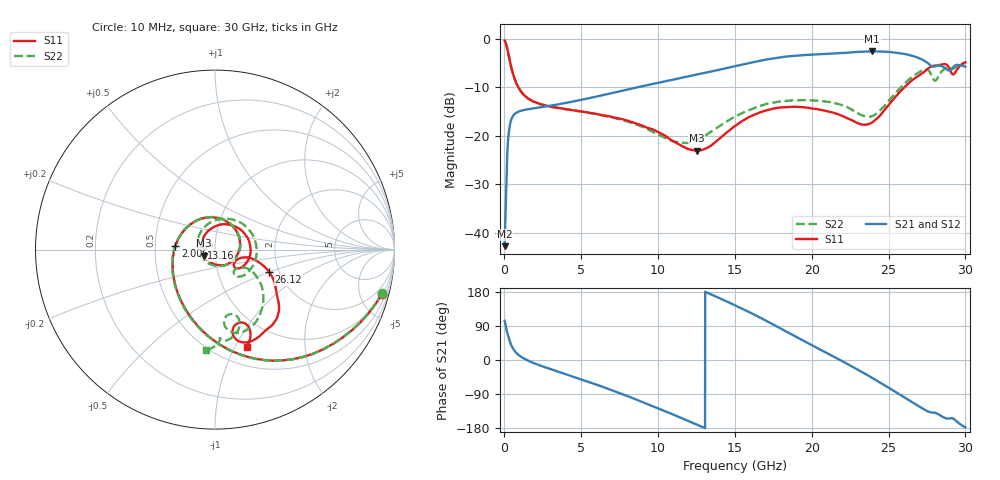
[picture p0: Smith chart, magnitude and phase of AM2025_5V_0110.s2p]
!Keysight Technologies,N5245B,MY58422270,A.16.20.02
!Date: Tuesday, July 14, 2026 01:05:04
!Correction: S11(C  2-Port  )
!S21(C  2-Port  )
!S12(C  2-Port  )
!S22(C  2-Port  )
!S2P File: Measurements: S11, S21, S12, S22:
# Hz S  dB  R 50
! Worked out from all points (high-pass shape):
!   3201 points, 10 MHz to 30 GHz, reference 50 ohm
!   highest |S21| = -2.59 dB at 23.94 GHz (marker M1); lowest = -42.8 dB at 10 MHz (marker M2)
!   |S21| within 3 dB of the highest: 15.09 GHz to 27.78 GHz (12.69 GHz wide, 59.2 % of centre); 29.28 GHz to 29.83 GHz (548.6 MHz wide, 1.86 % of centre)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
!   lowest |S11| = -23.1 dB at 12.5 GHz (marker M3), VSWR 1.15, Z = 44.1 - j3.06 ohm
!   |S11| at or under -10 dB: 904.8 MHz to 26.03 GHz (25.13 GHz wide, 187 % of centre)
!   |S22| runs from -21.5 to -0.3 dB; largest |S21 - S12| = 0.017
!   S11 on the Smith chart (normalised r, x): 10 MHz: 1.16, -7.56; 2.006 GHz: 0.64, +0.03; 13.16 GHz: 0.86, +0.02; 26.12 GHz: 1.77, -0.49; 30 GHz: 0.69, -1.12
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1e7  -0.34 -14.7  -42.79 103.5  -32.97 80.0  -0.34 -14.5
2.536688e8  -3.11 -62.2  -20.24 62.0  -20.22 62.0  -3.13 -62.6
4.317344e8  -5.75 -89.2  -16.79 40.3  -16.79 40.3  -5.77 -89.8
9.003281e8  -9.97 -131.1  -15.04 14.0  -15.04 14.0  -10.01 -132.3
2.006209e9  -13.09 174.5  -14.29 -9.7  -14.29 -9.7  -13.15 172.1
5.014581e9  -15.00 87.6  -12.58 -51.3  -12.57 -51.4  -15.01 82.2
7.535616e9  -16.48 24.5  -10.81 -88.0  -10.81 -88.0  -16.64 16.5
1.000979e10  -19.25 -44.6  -9.07 -127.4  -9.08 -127.5  -19.75 -59.0
1.250271e10  -23.08 -150.6  -7.38 -170.0  -7.37 -170.1  -20.92 -167.2
1.315874e10  -22.54 172.9  -6.94 178.3  -6.93 178.2  -19.78 163.2
1.5005e10  -17.99 93.4  -5.65 144.3  -5.65 144.3  -16.04 95.3
1.776033e10  -14.26 18.3  -3.90 87.8  -3.90 87.8  -13.01 23.9
2.000958e10  -14.37 -20.8  -3.26 39.1  -3.26 39.0  -12.71 -17.8
2.209014e10  -16.07 -41.7  -2.91 -5.3  -2.91 -5.3  -13.82 -47.5
2.39364e10  -17.23 -22.9  -2.59 -47.2  -2.60 -47.2  -15.94 -39.9
2.500479e10  -13.66 -13.4  -2.70 -73.1  -2.70 -73.2  -12.82 -30.1
2.612004e10  -9.74 -22.4  -3.16 -100.7  -3.16 -100.8  -8.98 -41.2
2.732902e10  -6.78 -39.5  -4.52 -130.7  -4.52 -130.8  -6.35 -68.0
2.803191e10  -5.52 -55.5  -5.68 -139.4  -5.68 -139.5  -8.65 -76.9
2.899721e10  -6.41 -78.1  -6.55 -153.8  -6.54 -153.9  -5.94 -85.7
2.929711e10  -7.14 -68.4  -5.56 -157.3  -5.56 -157.6  -6.03 -86.8
3e10  -4.86 -72.1  -5.76 -177.3  -5.74 -177.6  -4.98 -95.1
